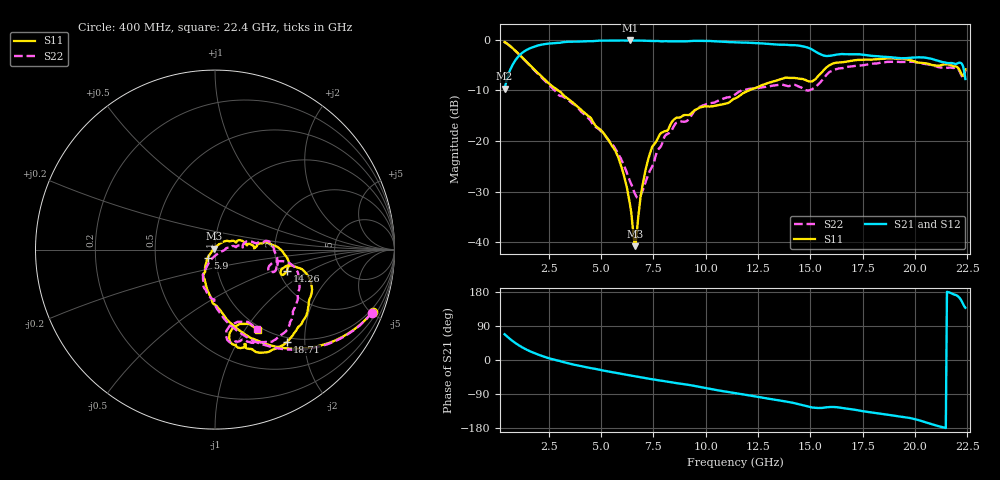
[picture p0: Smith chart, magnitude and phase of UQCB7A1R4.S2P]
!  Part Number  UQCB7A1R4	Mounting Orientation: Vertical
!  Description: RF capacitors
!  Application: Coupling, Bypass, Tuning, DC Block
!  Filters, Matching
# GHZ S DB R 50
! Freq  |S11|  S11 Ph  |S21|  S21 Ph  |S12|  S12 Ph  |S22|  S22 Ph
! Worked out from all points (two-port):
!   401 points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, 400 MHz to 22.4 GHz, reference 50 ohm
!   highest |S21| = -0.18 dB at 6.395 GHz (marker M1); lowest = -9.7 dB at 400 MHz (marker M2)
!   |S21| within 3 dB of the highest: 1.094 GHz to 15.65 GHz (14.55 GHz wide, 174 % of centre); 15.96 GHz to 17.84 GHz (1.87 GHz wide, 11.1 % of centre)
!   lowest |S11| = -40.8 dB at 6.615 GHz (marker M3), VSWR 1.02, Z = 49.3 + j0.525 ohm
!   |S11| at or under -10 dB: 2.938 GHz to 12.09 GHz (9.15 GHz wide, 122 % of centre)
!   |S22| runs from -31.3 to -0.5 dB; largest |S21 - S12| = 0.0054
!   S11 on the Smith chart (normalised r, x): 400 MHz: 0.80, -5.12; 5.9 GHz: 0.92, -0.09; 14.26 GHz: 2.20, -0.65; 18.71 GHz: 0.93, -1.66; 22.4 GHz: 0.95, -1.15
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0.4  -0.50 -21.6  -9.69 68.0  -9.70 68.0  -0.51 -21.9
1.005  -2.57 -47.7  -3.59 41.4  -3.60 41.4  -2.60 -48.6
1.885  -6.19 -71.4  -1.29 16.7  -1.30 16.7  -6.33 -73.5
4.085  -14.00 -104.9  -0.37 -16.6  -0.37 -16.6  -14.35 -110.0
5.24  -19.13 -119.7  -0.22 -29.2  -0.22 -29.2  -19.23 -116.2
5.9  -24.15 -131.7  -0.19 -35.8  -0.20 -35.8  -23.10 -113.5
6.395  -32.74 -146.4  -0.18 -40.7  -0.18 -40.7  -28.07 -97.0
6.615  -40.78 144.4  -0.18 -43.0  -0.18 -43.0  -30.36 -78.6
6.725  -37.55 85.5  -0.19 -44.1  -0.19 -44.1  -31.17 -64.2
6.835  -33.05 65.4  -0.20 -45.2  -0.20 -45.2  -31.14 -47.1
7.165  -25.15 46.3  -0.24 -48.5  -0.24 -48.4  -27.69 -12.3
7.77  -19.06 26.1  -0.31 -53.9  -0.31 -53.9  -21.51 6.7
8.65  -15.39 11.9  -0.37 -61.4  -0.37 -61.3  -16.36 5.9
11.4  -11.62 7.4  -0.54 -87.4  -0.56 -87.4  -10.88 9.7
14.26  -7.58 -16.9  -1.11 -114.2  -1.11 -114.2  -8.94 -19.3
15.085  -8.26 -16.2  -1.98 -125.4  -1.98 -125.3  -9.82 -14.1
16.075  -4.73 -21.4  -3.12 -124.0  -3.11 -123.9  -6.06 -19.3
18.715  -3.70 -51.8  -3.45 -144.6  -3.42 -144.7  -4.42 -48.1
18.77  -3.70 -52.6  -3.48 -145.0  -3.45 -145.3  -4.41 -48.8
20.53  -4.71 -71.6  -3.60 -164.9  -3.57 -165.0  -4.86 -64.7
22.015  -5.44 -79.8  -4.70 169.4  -4.69 169.3  -5.65 -81.1
22.4  -5.89 -61.8  -7.79 137.8  -7.80 137.6  -6.00 -61.9
